FUNCTION_BLOCK TwoStateSwitch
VAR
	digitalInput : I_DigitalInput;
END_VAR

METHOD FB_init : BOOL
VAR_INPUT
	bInitRetains : BOOL; // if TRUE, the retain variables are initialized (warm start / cold start)
	bInCopyCode : BOOL;  // if TRUE, the instance afterwards gets moved into the copy code (online change)
	DigitalInput : I_DigitalInput;
END_VAR
this^.digitalInput := DigitalInput;
END_METHOD

PROPERTY PUBLIC IsOn : BOOL
GET
IsOn := digitalInput.State;
END_GET
END_PROPERTY

END_FUNCTION_BLOCK
